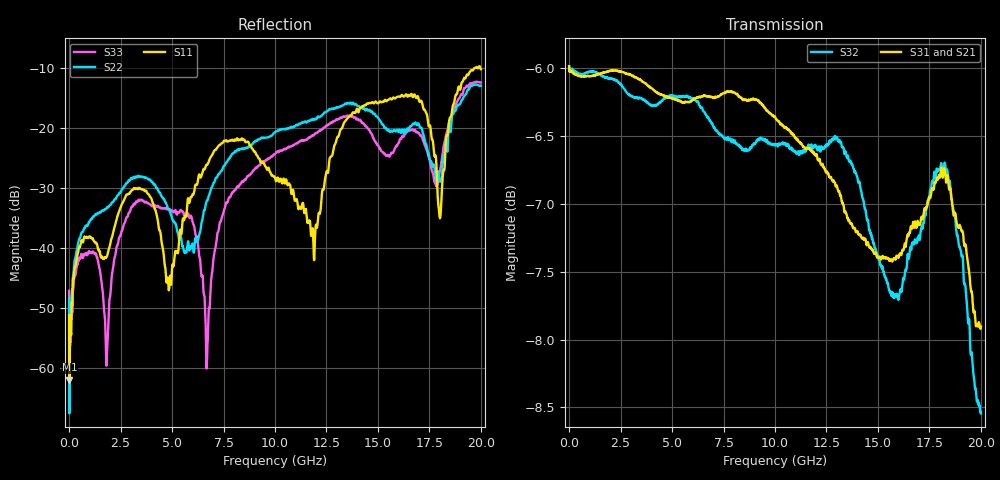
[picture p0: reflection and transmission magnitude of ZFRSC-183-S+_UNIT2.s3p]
!Mini-Circuits Laboratory
!S-Parameters
!Model: ZFRSC-183-S+
!Run/Lot/Date Code: F89730/NA/1038
!Fixture/SN/Due: NOT REQUIRED
!Connection: PORT 1 - SUM, PORT 2 - 1, PORT 3 - 2.
!Tested By: JIAN CHEN
!UNIT S/N: 2
!Agilent Technologies,N5230A,MY45001447,A.07.50.63
!Agilent N5230A: A.07.50.63
!Date: Wednesday, April 06, 2011 14:38:43
!Correction: S11(Full 3 Port(1,2,3))
!S12(Full 3 Port(1,2,3))
!S13(Full 3 Port(1,2,3))
!S21(Full 3 Port(1,2,3))
!S22(Full 3 Port(1,2,3))
!S23(Full 3 Port(1,2,3))
!S31(Full 3 Port(1,2,3))
!S32(Full 3 Port(1,2,3))
!S33(Full 3 Port(1,2,3))
!S3P File: Measurements: <S11,S12,S13>,
!<S21,S22,S23>,
!<S31,S32,S33>:
# Hz S  dB  R 50
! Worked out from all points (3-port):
!   2097 points, 300 kHz to 20 GHz, reference 50 ohm
!   strongest paths, dB at 300 kHz, 4.28 GHz, 9.52 GHz, 14.76 GHz, 20 GHz:
!     S31: -6.0, -6.2, -6.3, -7.3, -7.9
!     S21: -6.0, -6.3, -6.4, -7.2, -7.8
!     S32: -6.0, -6.3, -6.5, -7.3, -8.5
!   lowest |S11| = -61.9 dB at 12 MHz (marker M1), VSWR 1.00, Z = 49.9 + j0.0364 ohm
!   |S11| at or under -10 dB: start of sweep to 19.67 GHz; 19.97703 GHz to end of sweep
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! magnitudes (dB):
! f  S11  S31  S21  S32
! 300 kHz  -51.1  -6.0  -6.0  -6.0
! 12 MHz  -61.9  -6.0  -6.0  -6.0
! 1.1 GHz  -38.3  -6.1  -6.1  -6.0
! 1.82 GHz  -41.4  -6.0  -6.1  -6.1
! 5.85 GHz  -32.3  -6.2  -6.3  -6.2
! 6.71 GHz  -26.1  -6.2  -6.3  -6.4
! 10.01 GHz  -28.4  -6.4  -6.5  -6.6
! 16.7 GHz  -14.8  -7.1  -6.8  -7.3
! 18 GHz  -34.6  -6.8  -6.5  -6.7
! 20 GHz  -10.1  -7.9  -7.8  -8.5
